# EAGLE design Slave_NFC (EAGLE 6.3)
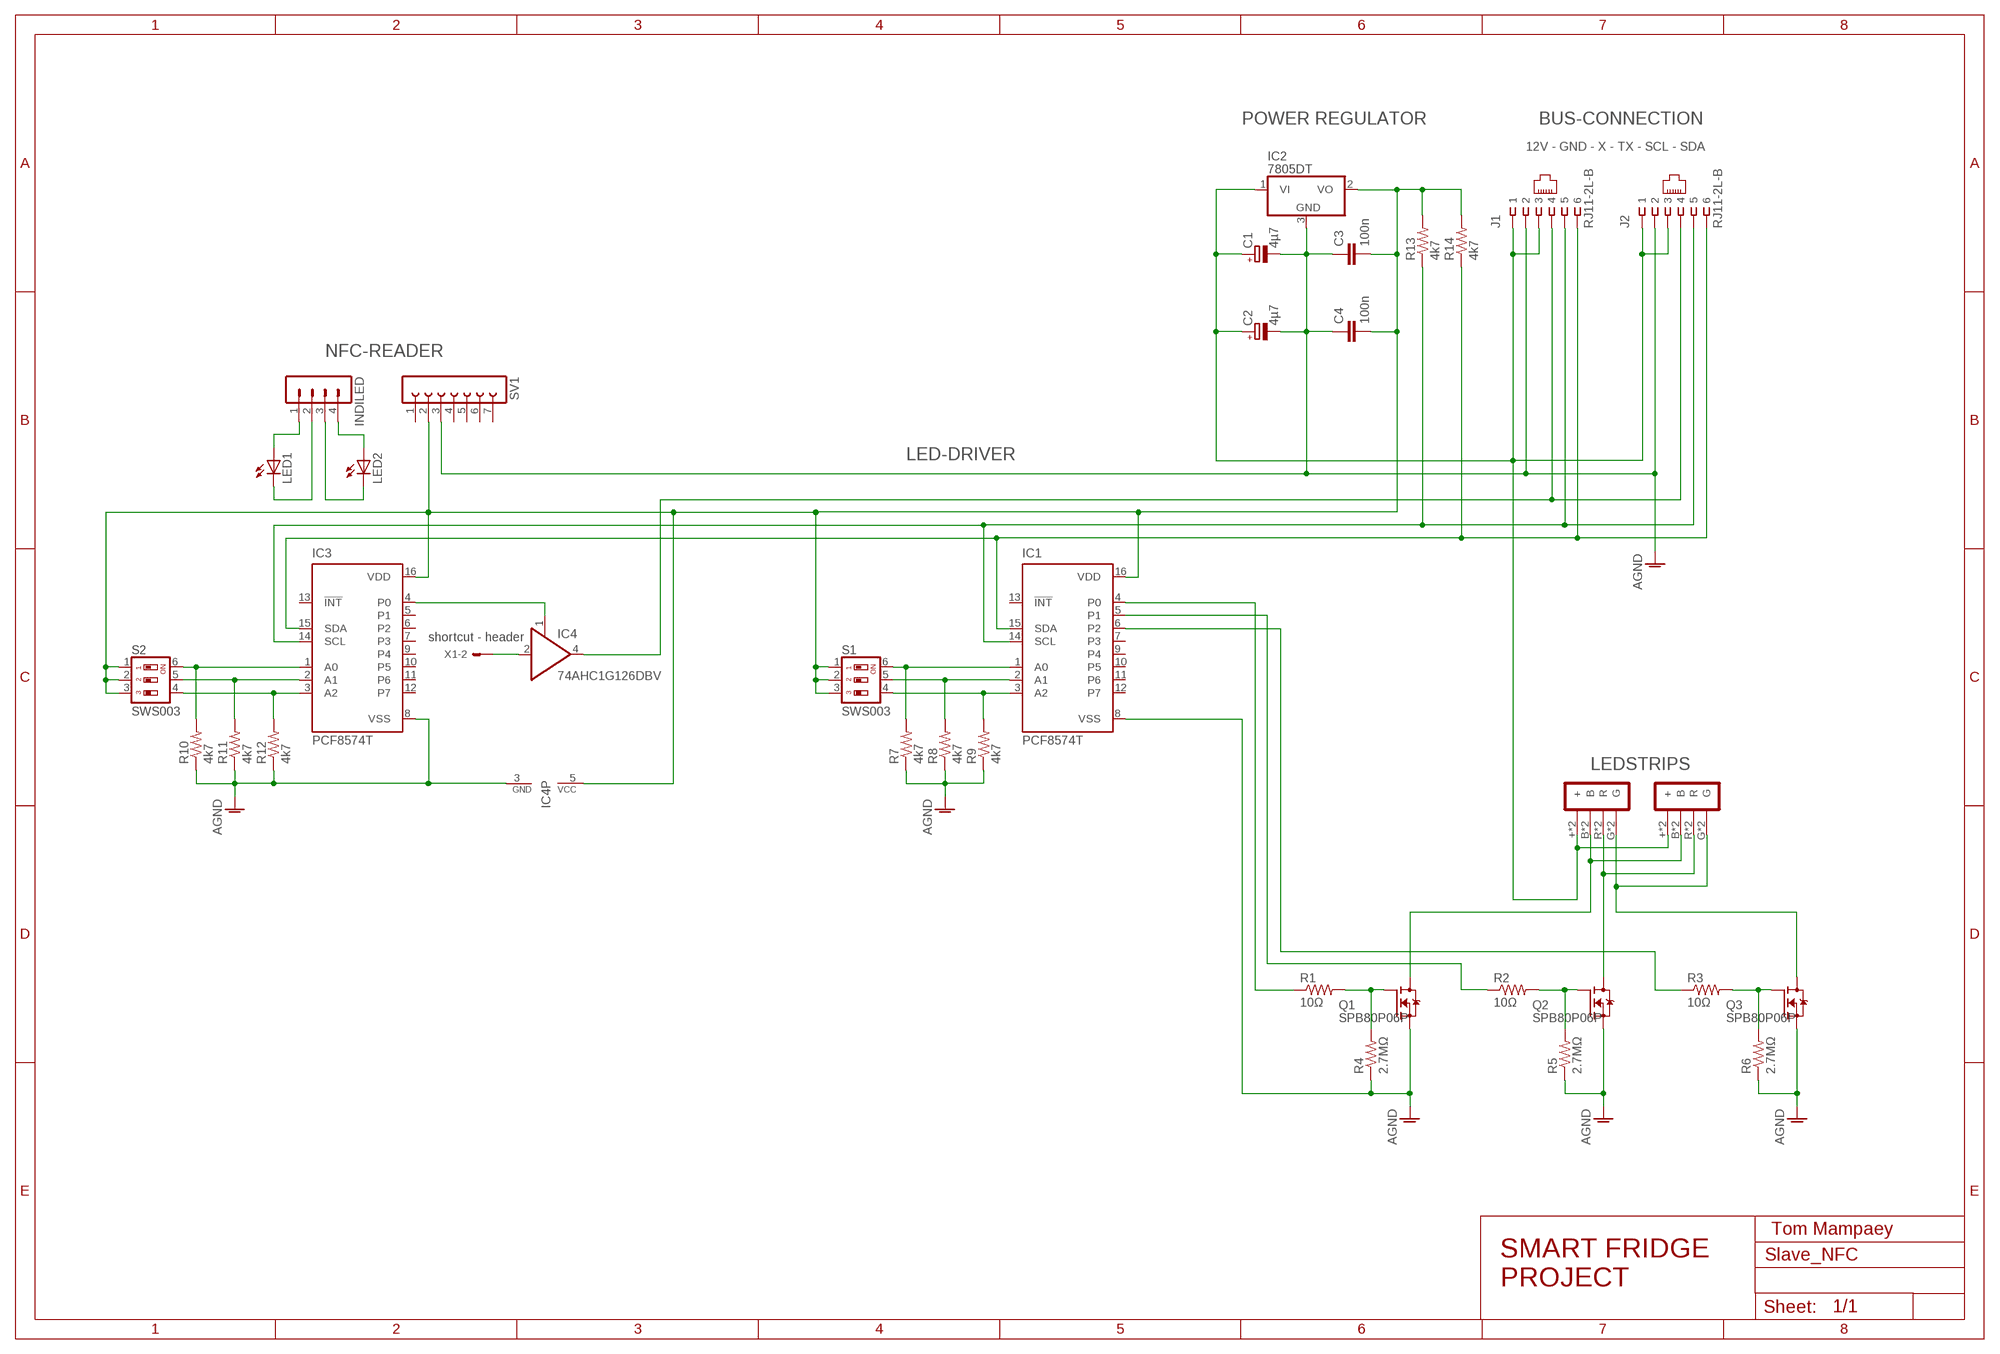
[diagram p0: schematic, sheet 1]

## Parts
C1  4µ7  CPOL-EUB  [PANASONIC_B]
C2  4µ7  CPOL-EUB  [PANASONIC_B]
C3  100n  C-EUC0603  [C0603]
C4  100n  C-EUC0603  [C0603]
IC1  PCF8574T  [SO16W]
IC2  7805DT  [TO252]
IC3  PCF8574T  [SO16W]
IC4  74AHC1G126DBV  [SOT23-5]
INDILED  MA04-1  [MA04-1]
J1  RJ11-2L-B  [RJ11-NO_SHIELD]
J2  RJ11-2L-B  [RJ11-NO_SHIELD]
LED1  LEDB152  [Q62902-B152]
LED2  LEDB152  [Q62902-B152]
Q1  SPB80P06P  [TO263]
Q2  SPB80P06P  [TO263]
Q3  SPB80P06P  [TO263]
R1  10Ω  R-US_R0402  [R0402]
R2  10Ω  R-US_R0402  [R0402]
R3  10Ω  R-US_R0402  [R0402]
R4  2.7MΩ  R-US_R0402  [R0402]
R5  2.7MΩ  R-US_R0402  [R0402]
R6  2.7MΩ  R-US_R0402  [R0402]
R7  4k7  R-US_R0402  [R0402]
R8  4k7  R-US_R0402  [R0402]
R9  4k7  R-US_R0402  [R0402]
R10  4k7  R-US_R0402  [R0402]
R11  4k7  R-US_R0402  [R0402]
R12  4k7  R-US_R0402  [R0402]
R13  4k7  R-US_R0402  [R0402]
R14  4k7  R-US_R0402  [R0402]
S1  SWS003  [SMS-003]
S2  SWS003  [SMS-003]
SV1  FE07-1  [FE07]
U$1  LED_S  [LED_P]
U$2  LED_S  [LED_P]
X1  22-23-2101  [22-23-2101]

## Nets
AGND: C1.- C2.- C3.1 C4.1 IC1.8(VSS) IC2.3(GND) IC3.8(VSS) IC4.3(GND) J1.2 J2.2 Q1.2(D) Q2.2(D) Q3.2(D) R4.1 R5.1 R6.1 R7.1 R8.1 R9.1 R10.1 R11.1 R12.1 SV1.3
N$1: IC1.15(SDA) IC3.15(SDA) J1.6 J2.6 R14.1
N$2: IC4.4(O) J1.4 J2.4
N$3: IC1.14(SCL) IC3.14(SCL) J1.5 J2.5 R13.1
N$4: Q1.1(G) R1.2 R4.2
N$5: Q2.1(G) R2.2 R5.2
N$6: Q3.1(G) R3.2 R6.2
N$7: Q1.3(S) U$1.B U$1.B1(B) U$2.B U$2.B1(B)
N$8: Q2.3(S) U$1.R U$1.R1(R) U$2.R U$2.R1(R)
N$9: Q3.3(S) U$1.G U$1.G1(G) U$2.G U$2.G1(G)
N$10: C1.+ C2.+ IC2.1(VI) J1.1 J1.3 J2.1 J2.3 U$1.+ U$1.+1(+) U$2.+ U$2.+1(+)
N$11: IC3.1(A0) R10.2 S2.6
N$12: IC1.1(A0) R7.2 S1.6
N$13: IC1.2(A1) R8.2 S1.5
N$14: IC1.3(A2) R9.2 S1.4
N$15: IC3.4(P0) IC4.1(OE)
N$16: IC1.4(P0) R1.1
N$17: IC1.5(P1) R2.1
N$18: IC1.6(P2) R3.1
N$19: IC3.2(A1) R11.2 S2.5
N$20: IC3.3(A2) R12.2 S2.4
N$21: C3.2 C4.2 IC1.16(VDD) IC2.2(VO) IC3.16(VDD) IC4.5(VCC) R13.2 R14.2 S1.1 S1.2 S1.3 S2.1 S2.2 S2.3 SV1.2
N$22: INDILED.1 LED1.A
N$23: INDILED.4 LED2.A
N$24: INDILED.2 LED1.K(C)
N$25: INDILED.3 LED2.K(C)
N$26: IC4.2(I) X1.2
Unconnected: IC1.7(P3) IC1.9(P4) IC1.10(P5) IC1.11(P6) IC1.12(P7) IC1.13(!INT) IC3.5(P1) IC3.6(P2) IC3.7(P3) IC3.9(P4) IC3.10(P5) IC3.11(P6) IC3.12(P7) IC3.13(!INT) SV1.1 SV1.4 SV1.5 SV1.6 SV1.7 X1.1 X1.3 X1.4 X1.5 X1.6 X1.7 X1.8 X1.9 X1.10

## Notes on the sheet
- POWER REGULATOR | BUS-CONNECTION
- 12V - GND - X - TX - SCL - SDA
- NFC-READER
- LED-DRIVER
- shortcut - header
- LEDSTRIPS
- Tom Mampaey
- SMART FRIDGE
  PROJECT

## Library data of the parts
C1 C2 = resistor:CPOL-EU: POLARIZED CAPACITOR, European symbol
C3 C4 = resistor:C-EU: CAPACITOR, European symbol
IC1 IC3 = micro-philips:PCF8574: I2C-Bus Remote 8-bit I/O expander http://www.semiconductors.philips.com/acrobat_download/datasheets/PCF8574_4.pdf; MPN: PCF8574T/3,512; OC_FARNELL: 1201255; OC_NEWARK: 70R6870
IC2 = linear:78*: Positive VOLTAGE REGULATOR Source: http://cache.national.com/ds/LM/LM78L05.pdf http://www.fairchildsemi.com/ds/LM/LM7805.pdf
IC4 = 74xx-little-de:74*1G126: Single Bus Buffer Gate With 3-State Outputs
INDILED = con-lstb:MA04-1: PIN HEADER; OC_FARNELL: unknown; OC_NEWARK: unknown
J1 J2 = con-tycoelectronics:RJ11: CORCOM Modular RJ Jacks No Shield Source: www.tycoelectronics.com .. ENG_DS_1654001_1099_RJ_L_0507.pdf; MF: TYCO ELECTRONICS; MPN: RJ11-2L-B; OC_FARNELL: unknown; OC_NEWARK: 83F4463
LED1 LED2 = led:LED: LED
Q1-Q3 = F3205S:SPB80P06P: SIPMOS (R) Power-Transistor P-Channel, Enhancement mode Source: http://www.infineon.com/upload/Document/cmc_upload/documents/011/3685/SPP80P06P.pdf
R1-R14 = rcl:R-US_: RESISTOR, American symbol
S1 S2 = smd-special:SWS003: SMD Dip Switch 3 pol.
SV1 = con-lsta:FE07-1: FEMALE HEADER; OC_FARNELL: unknown; OC_NEWARK: unknown
U$1 U$2 = Onboard_LEDstrip:LED_S
X1 = con-molex:22-23-2101: .100" (2.54mm) Center Header - 10 Pin; MF: MOLEX; MPN: 22-23-2101; OC_FARNELL: 1756828; OC_NEWARK: 94C0765

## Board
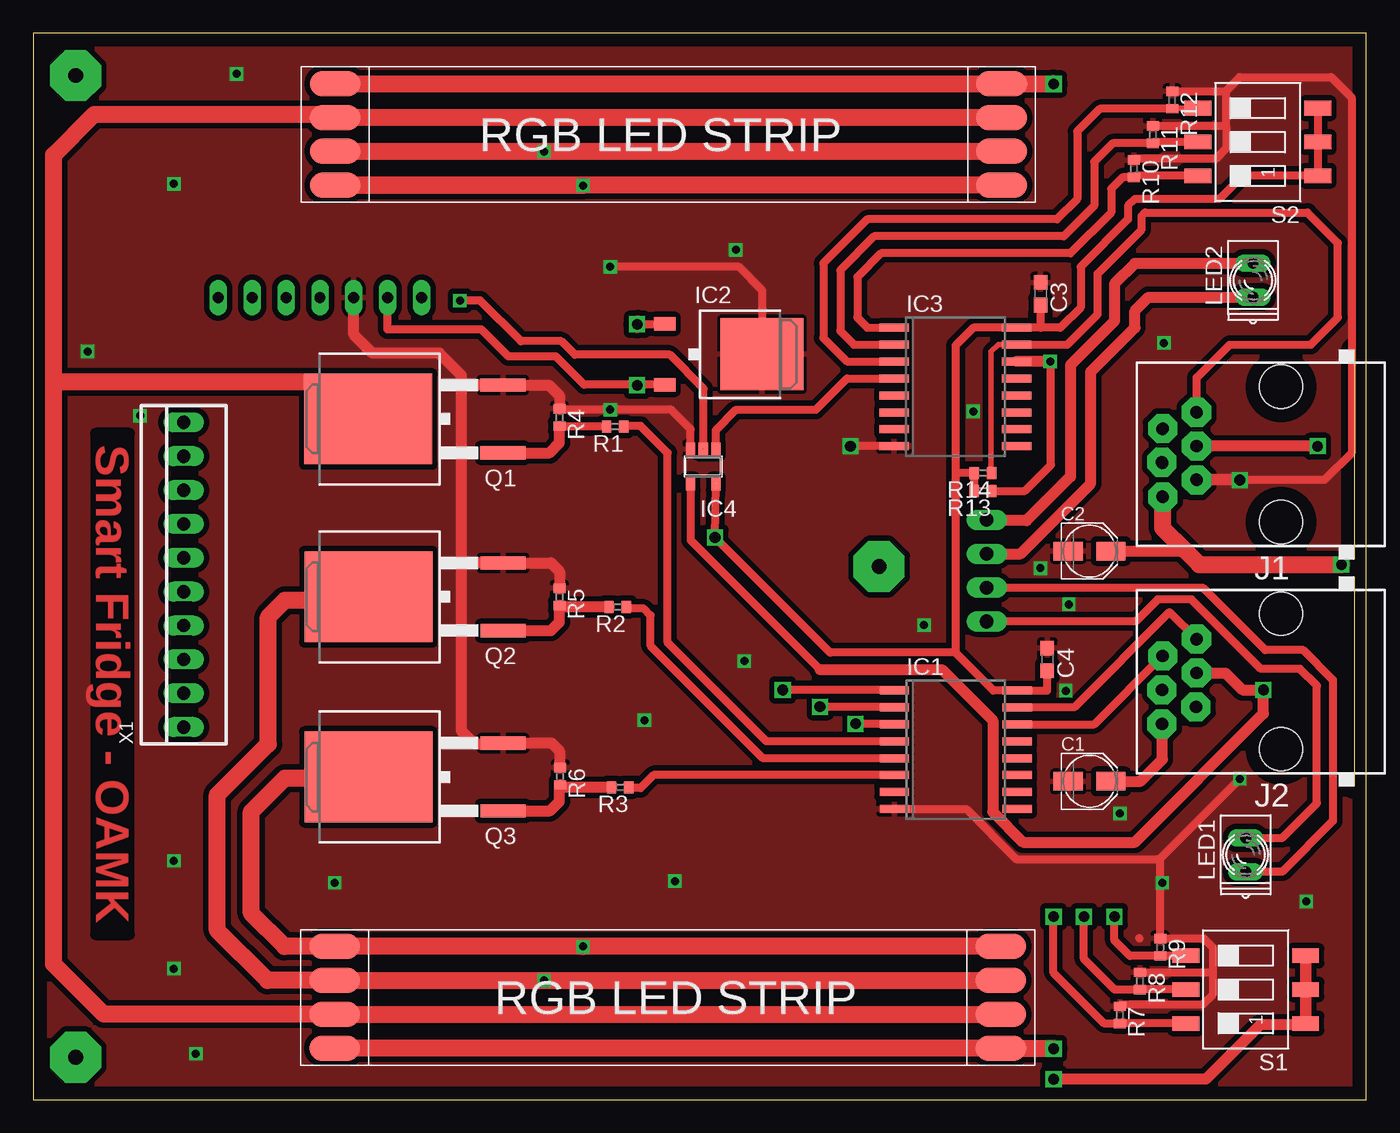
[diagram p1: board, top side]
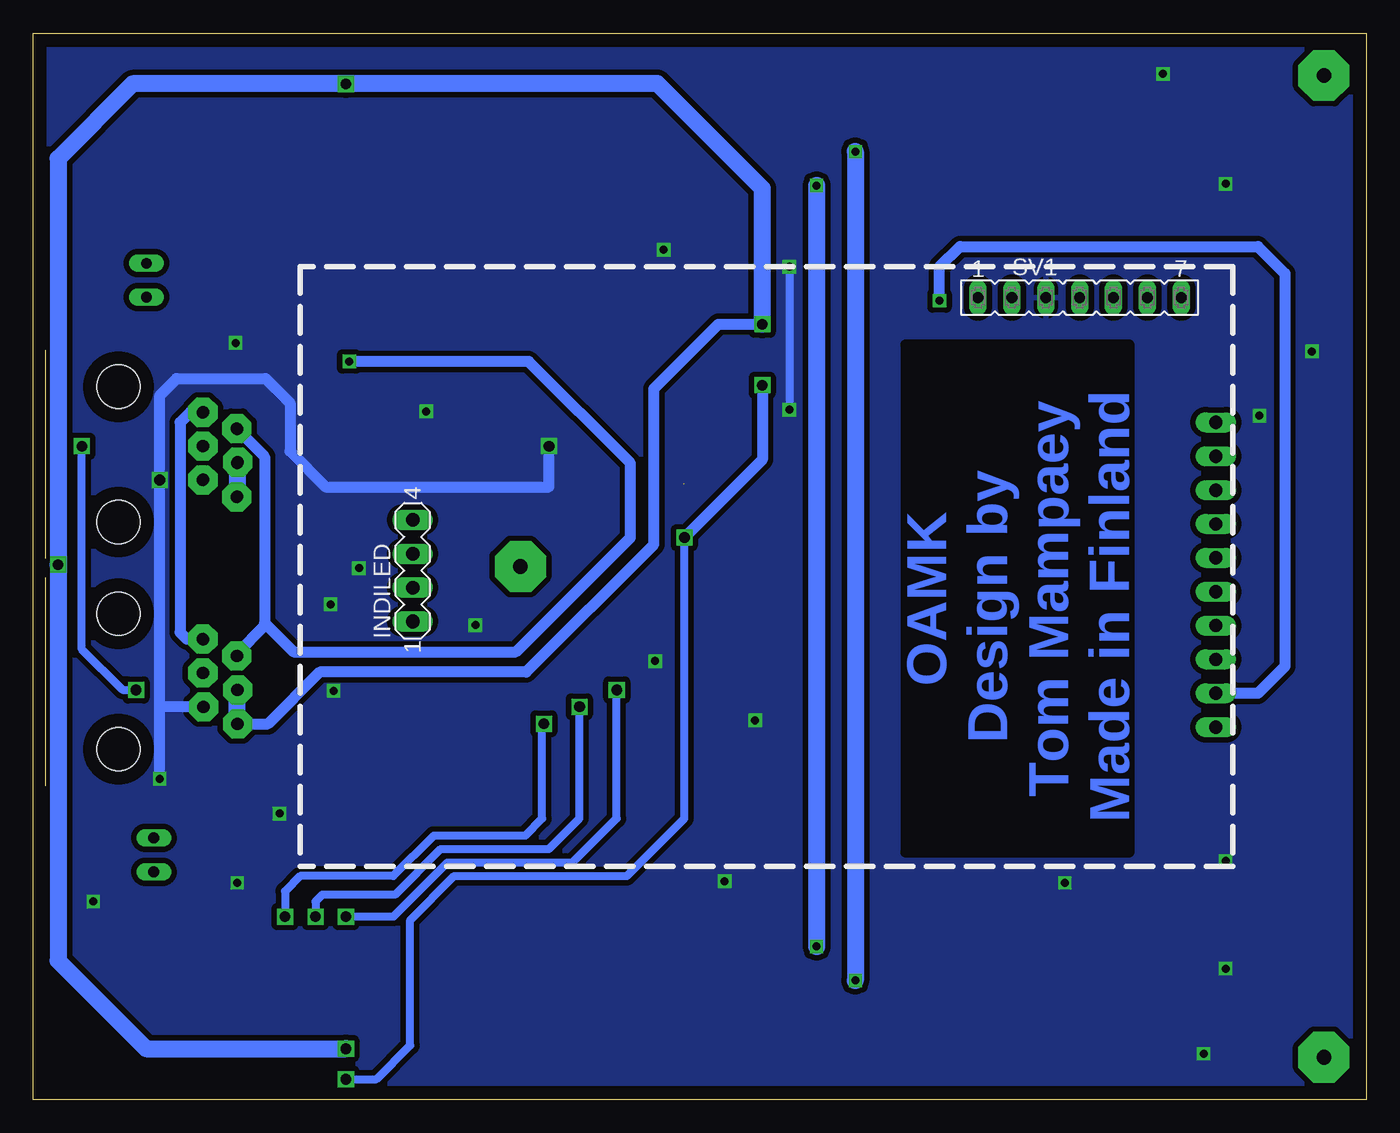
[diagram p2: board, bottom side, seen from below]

Size 100 x 80 mm. Coordinates in mm from the lower left corner, seen from the top.
Outline: 0,0 100,0 100,80 0,80 0,0
Copper layers (1*16): Top 0.035mm / dielectric 1.5mm / Bottom 0.035mm
Design rules "default": minimum track width 10mil, minimum drill 24mil, track to track 8mil, track to pad 8mil, pad to pad 8mil, via to via 8mil, smd to smd 8mil, copper to edge 40mil, drill to drill 8mil, minimum pad ring 10mil, minimum via ring 8mil, stop-mask expansion 4mil, vias tented up to drill 0mil, thermal gap 10mil

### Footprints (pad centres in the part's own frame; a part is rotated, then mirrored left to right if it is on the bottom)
PANASONIC_B = smd 2.2 x 1.4: + 1.6,0; - -1.6,0
C0603 = smd 1.1 x 1: 1 -0.85,0; 2 0.85,0
SO16W = smd 0.6 x 2.2: 1 -4.445,-4.6; 2 -3.175,-4.6; 3 -1.905,-4.6; 4 -0.635,-4.6; 5 0.635,-4.6; 6 1.905,-4.6; 7 3.175,-4.6; 8 4.445,-4.6; 9 4.445,4.6; 10 3.175,4.6; 11 1.905,4.6; 12 0.635,4.6; 13 -0.635,4.6; 14 -1.905,4.6; 15 -3.175,4.6; 16 -4.445,4.6
TO252 = smd 1 x 1.6: 1 -2.28,-4.8; 2 2.28,-4.8 | smd 5.4 x 6.2: 3 0,2.5
SOT23-5 = smd 0.69 x 0.99: 1 -0.95,-1.29; 2 0,-1.29; 3 0.95,-1.29; 4 0.95,1.3; 5 -0.95,1.3
MA04-1 = drill 1.016 long: 1 -3.81,0; 2 -1.27,0; 3 1.27,0; 4 3.81,0
RJ11-NO_SHIELD = drill 0.9 pad 1.4: 1 -3.175,8.89; 2 -1.905,6.35; 3 -0.635,8.89; 4 0.635,6.35; 5 1.905,8.89; 6 3.175,6.35 | hole 3.251: -5.08,0; 5.08,0
Q62902-B152 = drill 0.813 long: A 1.27,0; K -1.27,0
TO263 = smd 1 x 3.4: 1 -2.54,-6.6; 2 2.54,-6.6 | smd 6.8 x 9.6: 3 0,3.5
R0402 = smd 0.7 x 0.9: 1 -0.65,0; 2 0.65,0
SMS-003 = smd 1.092 x 2.007: 1 -2.54,-4.496; 2 0,-4.496; 3 2.54,-4.496; 4 2.54,4.496; 5 0,4.496; 6 -2.54,4.496
FE07 = drill 0.813 long: 1 -7.62,0; 2 -5.08,0; 3 -2.54,0; 4 0,0; 5 2.54,0; 6 5.08,0; 7 7.62,0
LED_P = smd 3.81 x 1.93: + -24.13,3.81; +1 25.87,3.81; B -24.13,1.27; B1 25.87,1.27; G -24.13,-3.81; G1 25.87,-3.81; R -24.13,-1.27; R1 25.87,-1.27
22-23-2101 = drill 1 long: 1 -11.43,0; 2 -8.89,0; 3 -6.35,0; 4 -3.81,0; 5 -1.27,0; 6 1.27,0; 7 3.81,0; 8 6.35,0; 9 8.89,0; 10 11.43,0

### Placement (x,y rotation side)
C1  79.25,23.88 0 top
C2  79.25,41.15 0 top
C3  75.56,60.45 270 top
C4  76.07,33.02 270 top
IC1  69.2,26.25 270 top
IC2  52.17,55.91 270 top
IC3  69.18,53.47 270 top
IC4  50.26,47.5 180 top
INDILED  71.54,39.68 90 bottom
J1  93.61,48.41 90 top
J2  93.61,31.36 90 top
LED1  90.96,18.36 90 top
LED2  91.51,61.47 90 top
Q1  28.63,51.06 90 top
Q2  28.64,37.72 90 top
Q3  28.64,24.2 90 top
R1  43.66,50.48 180 top
R2  43.85,36.96 180 top
R3  44.04,23.43 180 top
R4  39.46,51.18 270 top
R5  39.46,37.72 270 top
R6  39.53,24.26 270 top
R7  81.5,6.35 270 top
R8  83.03,8.89 270 top
R9  84.55,11.43 270 top
R10  82.58,69.85 270 top
R11  83.98,72.39 270 top
R12  85.44,74.99 270 top
R13  71.25,45.66 180 top
R14  71.25,47.02 180 top
S1  90.96,8.26 90 top
S2  91.87,71.84 90 top
SV1  21.5,60.17 0 bottom
U$1  46.78,72.42 0 top
U$2  48.47,7.67 180 top
X1  11.28,39.37 90 top

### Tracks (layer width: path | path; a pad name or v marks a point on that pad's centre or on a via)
AGND  (via drill 0.6, 0.8)
  Top 0.406: 82.58,70.61 R10.1
  Top 0.61: R12.1 89.3,75.64 89.5,75.44 | 89.5,73.04 R11.1 | 89.5,73.04 89.5,71.37 88.74,70.61 82.69,70.61 R10.1 | 89.5,73.04 89.5,75.44 | v90.52,46.48 96.87,46.48 98.9,48.51 98.9,75.18 97.38,76.71 90.52,76.71 89.5,75.69 89.5,75.44 | 88.49,9.4 88.49,11.43 87.84,12.08 R9.1 84.55,17.84 84.36,18.03 | 88.49,9.4 88.49,7.87 87.72,7.11 81.61,7.11 R7.1 | R8.1 88.34,9.54 88.49,9.4 | 83.01,12.08 82.96,12.13 | IC4.3 49.31,50.29 47.85,51.75 v43.27,51.75 39.54,51.75 R4.1 | IC1.8 69.99,21.8 73.75,18.03 84.49,18.03 v90.52,24.07 | IC2.3 54.7,55.91 54.7,60.71 52.93,62.48 v43.27,62.48 | IC3.8 v61.31,49.02
  Top 0.813: R6.1 39.46,24.97 39.46,26.16 38.88,26.74 Q3.2 35.17,26.67 33.11,26.67 32.1,27.69 32.1,40.13 | R5.1 39.46,39.62 38.83,40.26 Q2.2 32.23,40.26 32.1,40.13 | R4.1 39.46,52.83 38.69,53.6 Q1.2 32.11,53.6 32.1,52.83 | 32.1,52.83 32.1,40.13 | 32.1,52.83 32.1,54.36 30.45,56.01 25.43,56.01 24.03,57.4 SV1.3 | IC2.3 54.96,56.21 | v90.52,46.48 87.28,46.48 | v90.5,46.51 J1.2
  Bottom 0.61: v43.27,62.48 v43.27,51.75
  Bottom 0.813: 90.52,29.46 v90.52,46.48 | J2.2 90.51,29.45 90.52,29.46 | v90.5,46.51 v90.52,46.48 | v90.52,46.48 90.52,52.83 89.25,54.1 82.58,54.1 80.74,52.26 80.74,48.64 78.07,45.97 61.31,45.97 v61.31,49.02 | v90.52,24.07 90.52,29.46
  other vias: 22.61,16.26 12.19,3.43 48.13,16.38 45.85,28.45 53.34,32.89 84.84,56.77 66.83,35.59 10.54,68.71 15.24,76.96 95.5,14.86 52.7,63.75 10.54,17.91 84.71,16.26 70.52,51.63 4.06,56.13 8,51.31 81.53,21.46 75.56,39.88 77.47,30.67 77.69,37.15 10.54,9.81
  pour Bottom (isolate 0.406): 0,80.01 99.98,80.01 99.98,0 0,0
  pour Top (isolate 0.406): 0,80.01 99.92,80.01 99.92,0 0,0
N$1  (via drill 0.9 pad 2.18)
  Top 0.406: R14.1 71.85,47.02 71.85,56.1 72.39,56.64 IC3.15
  Top 0.61: IC3.15 77.56,56.64 79.85,58.93 79.85,61.98 83.15,65.28 83.15,66.29 83.41,66.55 95.6,66.55 97.88,64.26 97.88,58.67 95.85,56.64 89.76,56.64 87.28,54.17 87.28,51.56 J1.6 | v87.27,34.54 J2.6 | v87.28,34.54 85.25,36.58 78.09,29.42 IC1.15
  Bottom 0.813: J2.6 v87.27,34.54 v87.28,34.54 88.49,34.54 88.99,35.05 88.99,50.8 88.21,51.59 J1.6
N$2  (via drill 0.8, 0.9 pad 2.18)
  Top 0.61: IC4.4 49.31,41.97 59.02,32.26
  Top 0.813: 59.02,32.26 68.17,32.26 71.98,28.45 71.98,21.59 74.26,19.3 82.64,19.3 92.3,28.96 v92.3,30.73 90.71,30.73 89.44,32 v87.28,32 J2.4 | v96.36,49.02 87.28,49.02 J1.4
  Bottom 0.61: v96.36,49.02 96.36,33.78 93.31,30.73 v92.3,30.73
  Bottom 0.813: 87.28,49.02 J1.4
N$3  (via drill 0.6)
  Top 0.61: IC1.14 79.61,28.15 J2.5 | R13.1 74.39,45.66 76.36,47.62 76.36,55.31 v76.29,55.37
  Top 0.813: v76.29,55.37 IC3.14
  Bottom 0.813: J2.5 84.72,33.48 82.64,35.56 82.64,35.75 | J1.5 82.64,48.24 82.64,35.75 | 82.64,35.75 80.48,33.59 63.78,33.59 55.21,42.16 55.21,47.75 62.83,55.37 v76.29,55.37
N$4
  Top 0.61: R1.2 39.51,50.48
  Top 0.813: Q1.1 38.71,48.52 39.46,49.28 R4.2 39.51,50.48
N$5
  Top 0.813: Q2.1 38.83,35.18 39.46,35.81 R5.2 39.58,36.96 R2.2
N$6
  Top 0.813: Q3.1 38.77,21.66 39.46,22.35 39.46,23.54 R6.2 39.7,23.43 R3.2
N$7
  Top 1.27: U$2.B U$2.B1 5.29,6.4 1.52,10.16 1.52,53.66 | 22.07,73.69 U$1.B 23.21,73.69 | U$1.B1 23.21,73.69 | 23.21,73.69 22.98,73.91 4.57,73.91 1.52,70.87 1.52,53.66 | Q1.3 22.37,53.82 1.54,53.82 1.54,53.67 1.52,53.66
N$8  (via drill 0.6)
  Top 1.27: U$2.R 72.6,9.21 71.91,9.21 71.91,8.94 v38.32,8.94 U$2.R1 17.57,8.94 13.81,12.7 13.81,22.86 17.62,26.67 17.62,36.2 18.89,37.47 21.56,37.47 21.68,37.59 21.94,37.34 21.71,37.34 Q2.3 | U$1.R1 U$1.R 38.3,71.14 v38.32,71.12
  Bottom 1.27: v38.32,71.12 v38.32,8.94
N$9  (via drill 0.6)
  Top 1.27: U$2.G v41.24,11.48 U$2.G1 18.84,11.48 16.35,13.97 16.35,21.59 18.89,24.13 25.07,24.13 Q3.3 | U$1.G1 U$1.G 41.22,68.61 v41.24,68.58
  Bottom 1.27: v41.24,68.58 v41.24,11.48
N$10  (via drill 0.8)
  Top 0.61: 45.34,58.2 IC2.1
  Top 0.813: 84.84,28.07 J2.1 84.71,25.53 83.06,23.88 C1.+ | C2.+ 86.34,41.15 86.34,41.26
  Top 1.27: U$2.+1 U$2.+ 72.65,3.81 v76.55,3.81 | U$1.+ U$1.+1 76.52,76.22 v76.55,76.2 | J1.1 84.72,42.88 86.34,41.26 87.47,40.13 v98.14,40.13 | 45.34,58.2 v45.31,58.17
  Bottom 0.813: J2.1 82.4,28.18 78.52,32.07 63.02,32.07 53.43,41.66 53.43,53.34 48.61,58.17 v45.31,58.17
  Bottom 1.27: v76.55,3.81 91.53,3.81 98.14,10.41 v98.14,40.13 98.14,70.61 92.55,76.2 v76.55,76.2 76.52,76.22 53.18,76.22 45.31,68.35 v45.31,58.17 | J2.1 J2.3 | J1.3 J1.1
N$11
  Top 0.406: 82.58,69.3 R10.2
  Top 0.61: S2.6 82.68,69.3 R10.2 81.74,69.2 80.87,68.33 80.87,66.55 77.82,63.5 63.59,63.5 61.82,61.72 61.82,58.67 62.58,57.91 IC3.1
N$12  (via drill 0.8)
  Top 0.61: S1.6 81.52,5.71 R7.2 80.37,5.7 76.55,9.53 v76.55,13.72 | IC1.1 65.38,30.73 v56.23,30.73
  Bottom 0.61: v76.55,13.72 72.99,13.72 68.93,17.78 59.53,17.78 56.23,21.08 v56.23,30.73
N$13  (via drill 0.8)
  Top 0.61: S1.5 83.04,8.26 R8.2 81.14,8.24 78.83,10.54 v78.83,13.72 | IC1.2 65.38,29.46 v59.02,29.46
  Bottom 0.61: v78.83,13.72 78.83,14.86 78.33,15.37 72.86,15.37 69.44,18.8 61.31,18.8 59.02,21.08 v59.02,29.46
N$14  (via drill 0.8)
  Top 0.61: S1.4 84.56,10.79 R9.2 82.28,10.78 81.12,11.94 v81.12,13.72 | IC1.3 65.38,28.19 v61.69,28.19
  Bottom 0.61: v81.12,13.72 81.12,15.62 79.98,16.76 72.99,16.76 69.94,19.81 63.09,19.81 61.82,21.08 61.82,28.07 v61.69,28.19
N$15
  Top 0.61: IC4.1 51.21,50.23 52.74,51.75 58.7,51.75 61.05,54.1 IC3.4
N$16
  Top 0.61: IC1.4 55,26.88 47.59,34.29 47.59,48.51 45.56,50.55 44.37,50.55 R1.1
N$17
  Top 0.61: IC1.5 54.75,25.61 46.32,34.04 46.32,36.32 45.81,36.83 44.62,36.83 R2.1
N$18
  Top 0.61: IC1.6 46.53,24.34 45.56,23.37 44.75,23.37 R3.1
N$19
  Top 0.406: 83.98,71.84 R11.2
  Top 0.61: S2.5 84.08,71.84 R11.2 80.98,71.74 79.6,70.36 79.6,67.06 77.31,64.77 63.09,64.77 60.55,62.23 60.55,57.66 61.56,56.64 IC3.2
N$20
  Top 0.406: S2.4 85.44,74.38 R12.2
  Top 0.61: R12.2 80.03,74.34 78.33,72.64 78.33,67.56 76.8,66.04 62.58,66.04 59.28,62.74 59.28,57.15 61.05,55.37 IC3.3
N$21  (via drill 0.8)  (1 unrouted)
  Top 0.61: S2.3 S2.2 S2.1 90.73,69.3 88.99,67.56 82.64,67.56 82.14,67.06 82.14,66.04 78.58,62.48 78.58,59.44 77.06,57.91 75.56,57.91 | 75.56,57.91 IC3.16 70.52,57.91 69.18,56.58 69.18,46.99 | IC2.2 45.31,53.63 | 45.31,53.63 v45.31,53.59 | 45.31,53.63 41.33,53.63 39.21,55.75 35.65,55.75 33.62,57.78 26.57,57.78 SV1.2 | IC4.5 v51.15,42.16 59.78,33.53 69.18,33.53 | 69.18,33.53 72.02,30.69 IC1.16 76.07,30.69 C4.2 | 69.18,46.99 69.18,33.53 | C3.2 75.56,57.91 | 69.18,46.99 R14.2 R13.2
  Top 0.813: 45.35,53.63 v45.31,53.59 | S1.1 S1.2 S1.3 S1.1 95.6,5.59 92.04,5.59 87.98,1.52 v76.55,1.52
  Bottom 0.61: v76.55,1.52 74.26,1.52 71.72,4.06 71.72,13.46 68.42,16.76 55.47,16.76 51.15,21.08 v51.15,42.16
  Bottom 0.813: v45.31,53.59 45.31,48.01 v51.15,42.16
N$22
  Top 0.61: LED1.A 93.7,19.63 96.3,22.23 96.3,31.05 95.03,32.32 92.11,32.32 86.9,37.53 84.36,37.53 82.71,35.88 INDILED.1
N$23
  Top 0.813: LED2.A 82.64,62.74 81.12,61.21 81.12,58.42 77.82,55.12 77.82,46.74 74.52,43.43 71.6,43.43 INDILED.4
N$24
  Top 0.61: INDILED.2 87.73,38.41 92.42,33.72 95.28,33.72 97.5,31.5 97.5,20.89 93.69,17.08 LED1.K
N$25
  Top 0.813: INDILED.3 74.06,40.95 79.34,46.23 79.34,54.61 82.64,57.91 82.64,59.18 83.66,60.2 LED2.K
N$26  (via drill 0.6)
  Top 0.61: IC4.2 50.29,48.82 50.29,53.34 47.75,55.88 40.64,55.88 39.62,56.9 36.58,56.9 33.53,59.94 v32,59.94
  Bottom 0.813: v32,59.94 32,62.48 30.48,64.01 8.13,64.01 6.1,61.98 6.1,32.51 8.13,30.48 X1.2
N$28  (via drill 0.9 pad 2.18)
  other vias: 84.74,33.27
N$29  (via drill 0.9 pad 2.18)
  other vias: 84.68,30.73
N$30  (via drill 0.9 pad 2.18)
  other vias: 87.22,29.46
N$31  (via drill 0.9 pad 2.18)
  other vias: 84.68,28.19
N$32  (via drill 0.9 pad 2.18)
  other vias: 84.74,50.36
N$33  (via drill 0.9 pad 2.18)
  other vias: 84.68,47.82
N$34  (via drill 0.9 pad 2.18)
  other vias: 84.74,45.21
N$35  (via drill 0.9 pad 2.18)
  other vias: 87.28,46.48
N$36  (via drill 0.9 pad 2.18)
  other vias: 87.28,49.02
N$37  (via drill 0.9 pad 2.18)
  other vias: 87.28,51.56
N$38  (via drill 1.1 pad 3.81)
  other vias: 3.17,76.83
N$39  (via drill 1.1 pad 3.81)
  other vias: 3.17,3.17
N$40  (via drill 1.1 pad 3.81)
  other vias: 63.45,40

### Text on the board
Top: Smart Fridge - OAMK
Bottom: OAMK / Design by / Tom Mampaey / Made in Finland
